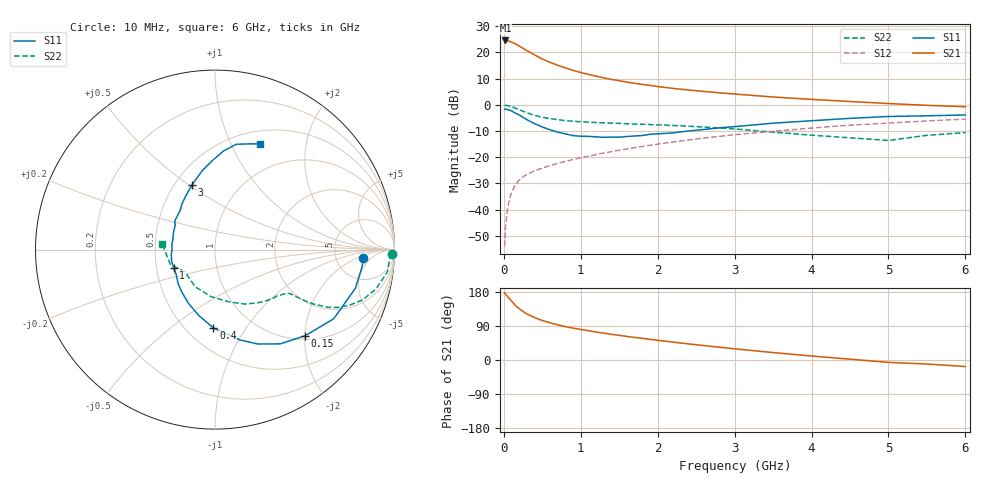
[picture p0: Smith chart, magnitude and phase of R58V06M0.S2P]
! SIEMENS Small Signal Semiconductors
! BFR183
! Si NPN RF Bipolar Junction Transistor in SOT23
! VCE = 8 V  IC = 6 mA
! Common Emitter S-Parameters:  May  1996
# GHz  S  MA  R  50
!  f  S11  S21  S12  S22
! GHz  MAG  ANG  MAG  ANG  MAG  ANG  MAG  ANG
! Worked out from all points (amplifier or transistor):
!   36 points, 10 MHz to 6 GHz, reference 50 ohm
!   highest |S21| = 24.6 dB at 20 MHz (marker M1)
!   |S21| within 3 dB of that: start of sweep to 248.2 MHz
!   unconditionally stable (mu >= 1): 1.002 GHz to 2.675 GHz
!   at 250 MHz: K = 0.46, MSG = 24.5 dB, |S12| = -27.5 dB
!   at 1.4 GHz: K = 1.06, MAG = 12.4 dB, |S12| = -17.9 dB
!   at 6 GHz: K = 0.88, MSG = 2.4 dB, |S12| = -5.5 dB
!   lowest NFmin = 1.20 dB at 450 MHz
!   S11 on the Smith chart (normalised r, x): 10 MHz: 10, -3; 150 MHz: 1.08, -2.01; 400 MHz: 0.67, -0.72; 1 GHz: 0.62, -0.13; 3 GHz: 0.61, +0.52; 6 GHz: 0.65, +1.30
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0.01  0.8267 -3.3  16.79 177.2  0.002 89.2  0.9853 -1.4
0.02  0.8257 -6.4  16.94 174.4  0.0043 87.7  0.9745 -2.9
0.05  0.8113 -15.4  16.79 167.1  0.0113 82.7  0.9688 -7.3
0.1  0.7657 -30.2  15.75 155.6  0.0212 75.6  0.9234 -13.8
0.15  0.6949 -43.7  14.62 144.0  0.0297 69.1  0.8663 -19.0
0.2  0.6389 -55.3  13.3 135.5  0.0366 65.0  0.8057 -22.8
0.25  0.577 -65.7  11.95 127.9  0.0422 62.0  0.7516 -25.4
0.3  0.5209 -74.8  10.83 121.5  0.0469 60.8  0.7048 -27.1
0.4  0.4364 -91.2  8.978 112.0  0.055 58.4  0.6286 -28.9
0.5  0.377 -104.1  7.493 104.2  0.0619 58.1  0.5774 -29.6
0.6  0.3339 -116.3  6.48 98.2  0.0693 58.0  0.5456 -29.9
0.8  0.2791 -137.6  5.061 88.1  0.0829 59.0  0.4997 -30.2
1  0.2512 -156.2  4.142 80.5  0.0974 60.0  0.4753 -30.9
1.1  0.2499 -165.4  3.811 77.3  0.1049 60.4  0.4664 -31.8
1.3  0.2394 -179.8  3.266 70.9  0.1203 60.3  0.4527 -33.2
1.6  0.2485 159.2  2.711 62.1  0.1439 60.0  0.4342 -36.4
2.2  0.2908 132.2  2.06 47.2  0.1952 57.3  0.4035 -44.9
3  0.3835 109.4  1.606 29.5  0.2687 50.5  0.3462 -61.2
3.5  0.4455 99.2  1.41 19.6  0.3128 45.0  0.3002 -75.5
4.5  0.5513 85.1  1.157 2.2  0.4091 33.6  0.2344 -118.2
5.5  0.6174 72.5  0.978 -10.6  0.4929 21.7  0.2615 -161.5
6  0.6399 67.0  0.918 -17.2  0.5327 13.9  0.295 174.4
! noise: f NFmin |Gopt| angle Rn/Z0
0.45  1.2  0.21  41  0.24
0.9  1.25  0.24  101  0.21
1.8  2  0.32  175  0.14
